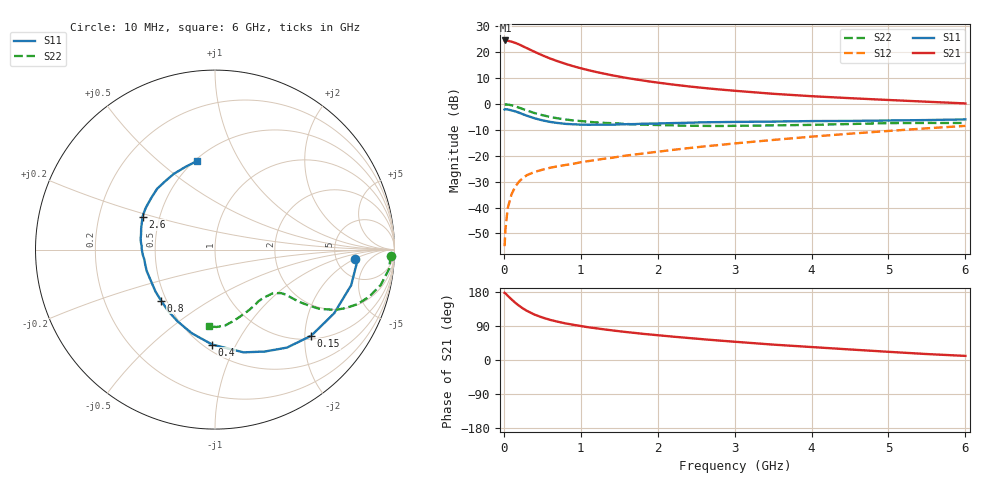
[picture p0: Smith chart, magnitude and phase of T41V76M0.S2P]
! Infineon Technologies  Discrete & RF Semiconductors
! BFR182T
! Si NPN RF Bipolar Junction Transistor in SC75
! VCE = 1.75 V  IC = 6 mA
! Common Emitter S-Parameters:  October  1999
# GHz  S  MA  R  50
!  f  S11  S21  S12  S22
! GHz  MAG  ANG  MAG  ANG  MAG  ANG  MAG  ANG
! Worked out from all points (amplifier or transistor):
!   36 points, 10 MHz to 6 GHz, reference 50 ohm
!   highest |S21| = 24.5 dB at 20 MHz (marker M1)
!   |S21| within 3 dB of that: start of sweep to 301 MHz
!   unconditionally stable (mu >= 1): 1.224 GHz to 3.982 GHz
!   at 250 MHz: K = 0.32, MSG = 25.4 dB, |S12| = -28.5 dB
!   at 1.4 GHz: K = 1.05, MAG = 14.6 dB, |S12| = -20.8 dB
!   at 6 GHz: K = 0.85, MSG = 4.3 dB, |S12| = -8.5 dB
!   lowest NFmin = 1.25 dB at 450 MHz
!   S11 on the Smith chart (normalised r, x): 10 MHz: 7.56, -2.12; 150 MHz: 1.08, -2.15; 400 MHz: 0.55, -0.81; 800 MHz: 0.47, -0.32; 2.6 GHz: 0.40, +0.18; 6 GHz: 0.51, +0.68
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0.01  0.7818 -4.0  16.72 177.2  0.0018 80.3  0.9806 -2.0
0.02  0.7955 -4.6  16.85 176.1  0.0037 95.9  0.9788 -2.5
0.05  0.7841 -14.7  16.63 169.6  0.0097 86.3  0.9764 -6.3
0.1  0.7528 -28.1  16 160.0  0.0181 77.6  0.9446 -12.0
0.15  0.7193 -41.9  15.1 150.8  0.0256 70.4  0.8984 -17.0
0.2  0.6774 -53.7  14.09 142.8  0.0321 66.8  0.8489 -21.0
0.25  0.632 -64.0  12.97 135.9  0.0374 62.7  0.7958 -24.2
0.3  0.5941 -74.5  11.95 129.7  0.0423 59.2  0.7507 -26.6
0.4  0.5292 -91.7  10.16 119.7  0.0488 55.8  0.6677 -29.6
0.5  0.4839 -105.4  8.714 112.2  0.0538 53.8  0.6091 -30.8
0.6  0.4512 -117.5  7.571 106.0  0.0587 52.9  0.5635 -31.6
0.7  0.4299 -127.6  6.688 101.1  0.0627 52.9  0.5288 -32.0
0.8  0.4134 -136.6  5.974 96.7  0.0664 53.4  0.5033 -32.2
1.1  0.3969 -157.8  4.497 86.3  0.079 55.9  0.454 -32.9
1.4  0.3978 -172.1  3.6 78.4  0.0912 57.5  0.4263 -34.7
1.6  0.4079 179.8  3.178 73.6  0.1015 58.9  0.4105 -36.0
2.2  0.4282 163.9  2.371 61.6  0.1302 61.5  0.3869 -42.4
2.6  0.4435 155.6  2.038 54.6  0.1513 62.3  0.378 -47.5
3.5  0.4576 140.6  1.574 40.6  0.2023 61.6  0.3864 -60.2
4.5  0.471 126.6  1.296 27.8  0.267 58.3  0.4106 -75.3
5.5  0.4896 109.6  1.106 15.7  0.3393 53.2  0.4311 -88.8
6  0.504 101.3  1.026 10.8  0.3779 49.5  0.4297 -94.5
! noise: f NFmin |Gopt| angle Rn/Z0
0.45  1.25  0.25  39  0.3
0.9  1.4  0.25  78  0.23
1.8  1.95  0.21  151  0.2
